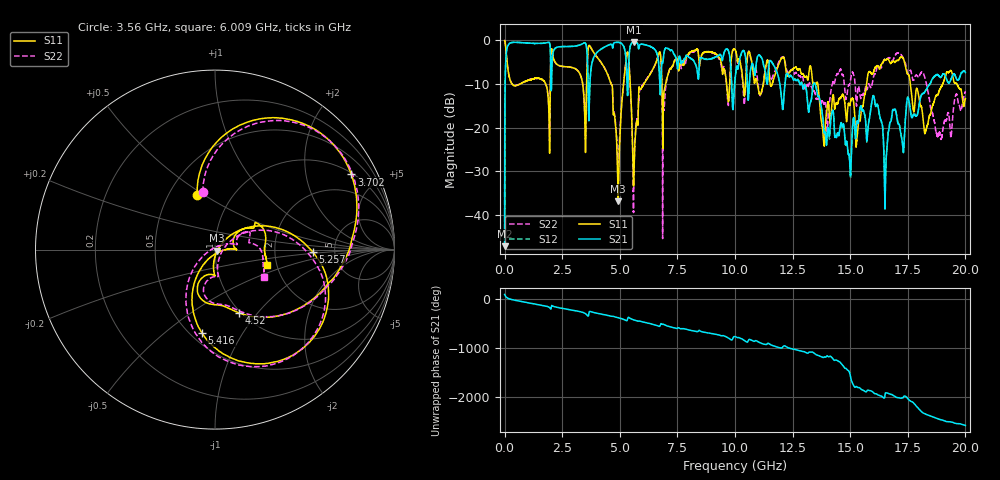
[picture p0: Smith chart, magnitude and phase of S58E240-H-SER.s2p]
!{S58E240}
!Johanson Technology Inc.
!www.johansontechnology.com
!Test Board Conditions:
!Substrate Type  RO4350B
!Substrate Thickness  60 mil
!Substrate Dk  3.66
!TL Type: GCPW
!TL Trace Width  115 mil
!TL Gap  52 mil
!Electrode orientation  Horizontal
!DUT TOPOLOGY	SERIES
!Mounting Pad LxW  55x428 mil
! Created Wed Apr 14 11:33:23 2021
# mhz S ma R 50
! 2 Port Network Data from SP1.SP block
! freq  magS11  angS11  magS21  angS21  magS12  angS12  magS22  angS22
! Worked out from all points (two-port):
!   20001 points, 300 kHz to 20 GHz, reference 50 ohm
!   highest |S21| = -0.39 dB at 5.617 GHz (marker M1); lowest = -47.2 dB at 300 kHz (marker M2)
!   |S21| within 3 dB of the highest: 65.36 MHz to 1.992 GHz (1.927 GHz wide, 187 % of centre); 2.084 GHz to 3.585 GHz (1.501 GHz wide, 53 % of centre)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
!   lowest |S11| = -36.9 dB at 4.931 GHz (marker M3), VSWR 1.03, Z = 51.3 - j0.647 ohm
!   |S11| at or under -10 dB: 5.454 GHz to 6.044 GHz (590.6 MHz wide, 10.3 % of centre); 13.59 GHz to 15.71 GHz (2.119 GHz wide, 14.5 % of centre); 17.61 GHz to 19.02 GHz (1.407 GHz wide, 7.68 % of centre)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
!   |S22| runs from -45.5 to 0.0 dB; largest |S21 - S12| = 0.013
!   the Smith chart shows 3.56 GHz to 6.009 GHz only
!   S11 on the Smith chart (normalised r, x): 3.56 GHz: 0.69, +0.47; 3.702 GHz: 1.06, +3.59; 4.52 GHz: 0.98, -0.80; 5.257 GHz: 3.38, -0.11; 5.416 GHz: 0.57, -0.68; 6.009 GHz: 1.78, -0.34
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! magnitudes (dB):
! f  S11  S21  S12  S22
! 300 kHz  0.0  -47.2  -47.2  0.0
! 103.3 MHz  -4.9  -1.8  -1.8  -4.8
! 193.3 MHz  -8.2  -0.8  -0.8  -8.2
! 3.334 GHz  -8.6  -0.9  -0.9  -8.6
! 3.56 GHz  -9.9  -1.7  -1.7  -9.7
! 3.702 GHz  -1.2  -10.0  -9.9  -1.2
! 4.52 GHz  -8.5  -1.0  -1.0  -8.5
! 4.931 GHz  -36.9  -0.4  -0.4  -28.0
! 5.257 GHz  -5.3  -3.6  -3.6  -5.3
! 5.416 GHz  -6.6  -2.7  -2.7  -6.6
! 5.617 GHz  -29.7  -0.4  -0.4  -30.0
! 6.009 GHz  -10.4  -0.9  -0.9  -10.1
! 6.667 GHz  -3.5  -4.4  -4.4  -3.5
! 6.923 GHz  -11.5  -2.7  -2.7  -15.7
! 10 GHz  -2.1  -8.9  -8.9  -2.1
! 13.33 GHz  -7.7  -12.9  -13.0  -10.8
! 13.83 GHz  -21.7  -18.5  -18.6  -14.2
! 15.31 GHz  -21.8  -18.5  -18.6  -12.5
! 16.67 GHz  -4.4  -20.8  -20.7  -4.0
! 18.28 GHz  -20.8  -11.4  -11.5  -9.2
! 18.88 GHz  -11.4  -8.3  -8.4  -21.1
! 20 GHz  -13.3  -7.3  -7.3  -11.9
